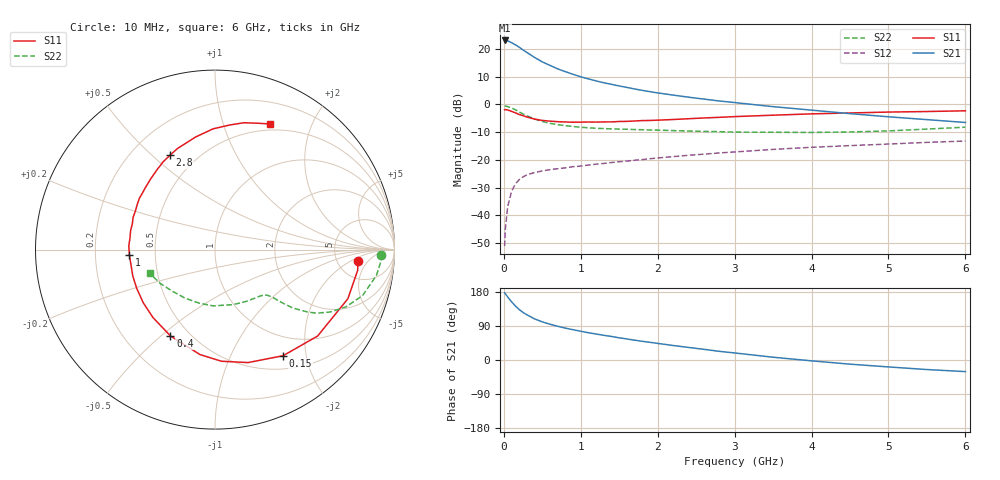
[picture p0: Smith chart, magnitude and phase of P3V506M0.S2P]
! SIEMENS Small Signal Semiconductors
! BFP181
! Si NPN RF Bipolar Junction Transistor in SOT143
! VCE = 0.5 V  IC = 6 mA
! Common Emitter S-Parameters:  March  1996
# GHz  S  MA  R  50
!  f  S11  S21  S12  S22
! GHz  MAG  ANG  MAG  ANG  MAG  ANG  MAG  ANG
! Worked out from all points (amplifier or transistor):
!   36 points, 10 MHz to 6 GHz, reference 50 ohm
!   highest |S21| = 23.0 dB at 10 MHz (marker M1)
!   |S21| within 3 dB of that: start of sweep to 228.2 MHz
!   unconditionally stable (mu >= 1): 676.2 MHz to end of sweep
!   at 250 MHz: K = 0.44, MSG = 22.8 dB, |S12| = -26.1 dB
!   at 1.4 GHz: K = 1.57, MAG = 9.6 dB, |S12| = -21.0 dB
!   at 6 GHz: K = 1.67, MAG = -1.5 dB, |S12| = -13.2 dB
!   S11 on the Smith chart (normalised r, x): 10 MHz: 7.93, -2.81; 150 MHz: 0.69, -1.61; 400 MHz: 0.40, -0.54; 1 GHz: 0.35, -0.03; 2.8 GHz: 0.36, +0.57; 6 GHz: 0.43, +1.44
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0.01  0.7987 -4.6  14.09 177.3  0.0028 86.7  0.9278 -1.7
0.02  0.8032 -8.3  14.08 174.9  0.0058 81.8  0.9279 -3.7
0.05  0.7893 -20.3  13.86 166.3  0.0144 80.4  0.911 -9.1
0.1  0.7475 -40.1  12.87 153.7  0.027 67.1  0.8611 -17.3
0.15  0.7025 -57.3  11.78 142.6  0.037 60.2  0.7965 -23.6
0.2  0.6558 -73.7  10.65 133.1  0.0441 53.9  0.7306 -28.4
0.25  0.6231 -86.7  9.481 125.3  0.0494 48.5  0.6685 -32.0
0.3  0.5906 -98.2  8.563 119.3  0.0539 45.0  0.6216 -34.0
0.4  0.5411 -117.3  6.969 108.5  0.0592 40.0  0.5449 -36.8
0.5  0.5125 -132.4  5.794 100.6  0.0633 36.7  0.49 -38.1
0.6  0.4975 -143.5  5.012 94.4  0.0667 35.2  0.4542 -38.9
0.8  0.481 -162.3  3.867 84.1  0.0719 34.2  0.4128 -39.8
1  0.4781 -176.7  3.124 75.8  0.0774 34.2  0.386 -41.2
1.1  0.4806 177.5  2.863 71.9  0.0808 34.3  0.3778 -42.2
1.3  0.4819 167.2  2.439 65.1  0.0863 34.3  0.3658 -44.5
1.7  0.5009 149.9  1.886 52.3  0.0985 34.3  0.3514 -49.9
2.2  0.5324 132.4  1.465 38.3  0.1144 33.2  0.3365 -59.2
2.8  0.5827 115.5  1.148 22.9  0.1332 30.3  0.3222 -72.7
3.5  0.6369 99.7  0.907 7.3  0.1544 26.1  0.3139 -91.4
4.5  0.6986 83.4  0.679 -11.0  0.1805 18.5  0.3179 -121.7
5.5  0.7415 71.8  0.53 -25.2  0.2064 11.5  0.3583 -148.2
6  0.764 66.4  0.471 -30.6  0.2184 7.4  0.3874 -160.1
